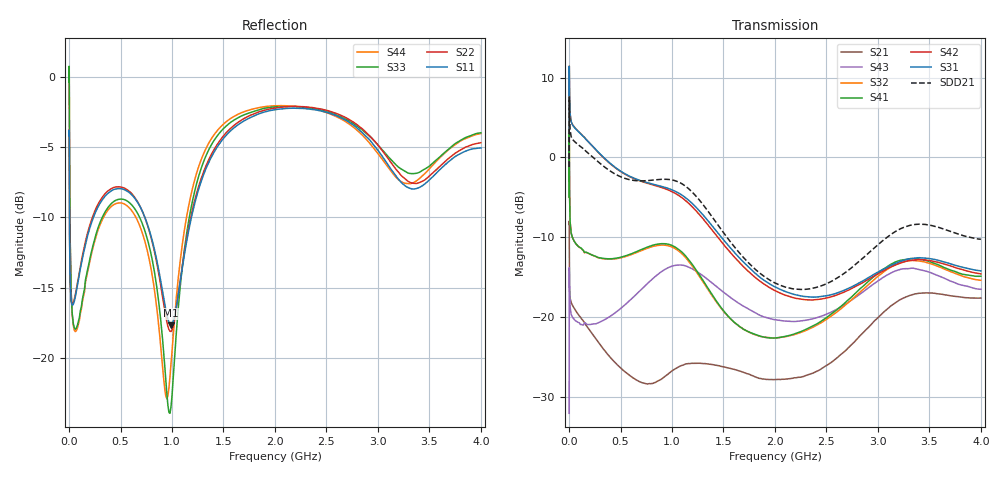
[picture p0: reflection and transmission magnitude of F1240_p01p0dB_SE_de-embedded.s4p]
! Integrated Device Technology
! Corporate Headquarters
! 6024 Silver Creek Valley Road
! San Jose, CA 95138  USA
! Phone:  1-408-284-8200
! Toll Free:  1-800-223-1366
! Webpage:  http://www.idt.com/
! Timing and RF Division
! 515 Groton Road, Suite 102
! Westford, MA 01886-6024
! Device:  F1240
! Description: Dual Intermediate Frequency Digital Variable Gain Amplifier
! Frequency:  10.0 -  500.00 MHz
! Package:  5x5 mm QFN Plastic Package: 32 pin
! Ports:  8 RF, 20 DC
!  Pin  1  = GA3 / Data  Pin 17  = RF OUT_B+
!  Pin  2  = GA4 / CLK  Pin 18  = RF OUT_B-
!  Pin  3  = GA5  Pin 19  = STBY_B
!  Pin  4  = VMODE  Pin 20  = Ground
!  Pin  5  = No Connect  Pin 21  = Ground
!  Pin  6  = GB5  Pin 22  = STB_A
!  Pin  7  = GB4  Pin 23  = RF OUT_A-  = Port 4
!  Pin  8  = GB3  Pin 24  = RF OUT_A+  = Port 3
!  Pin  9  = GB2  Pin 25  = GA0
!  Pin 10  = GB1  Pin 26  = ISET_A
!  Pin 11  = RF IN_B+  Pin 27  = VCC
!  Pin 12  = RF IN_B-  Pin 28  = Ground
!  Pin 13  = Ground  Pin 29  = RF IN_A-  = Port 2
!  Pin 14  = VCC  Pin 30  = RF IN_A+  = Port 1
!  Pin 15  = ISET_B  Pin 31  = GA1
!  Pin 16  = GB0  Pin 32  = GA2 / CSb
! Gain  = +19.5 dB
! State  = 1
! Voltage  = +5.00 V
! Current  = 85.292 mA (one channel only)
! Temperture  =  +25 C
! Test Date  =  2017-10-18
! Board  =  EB4031
! Data:  The device was measured on a custom evaluation board which has
!  individual transmission lines to the RF pins.  Data was collected
!  using a calibrated network analyzer.  The evaluation board was
!  de-embedded using Automatic Fixture Removal.
!  The reference plane is the edge of the package pin.
!  Only Channel A was measured.
!  This data is in single-ended operation.  If your needs are balanced
!  or differential S-parameters then this file needs to be used a
!  linear simulator.
! File Date:  2017-11-10  MJV
! Note:
!  Integrated Device Technology supplies this data as a sample of measured
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# Hz S dB R 100
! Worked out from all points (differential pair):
!   410 points, 500 kHz to 4 GHz, reference 100 ohm
!   strongest paths, dB at 500 kHz, 930 MHz, 1.96 GHz, 2.98 GHz, 4 GHz:
!     S31: 3.1, -3.7, -15.9, -14.5, -14.2
!     S42: 3.1, -3.9, -16.4, -14.7, -14.6
!     S41: -5.0, -10.8, -22.6, -14.7, -14.9
!     S32: -5.0, -11.0, -22.6, -15.1, -15.4
!     S43: -32.0, -14.0, -20.2, -15.7, -16.5
!     S21: -8.4, -27.4, -27.8, -20.3, -17.6
!   taken as a pair (ports 1,2 in; 3,4 out), SDD21 dB: -1.2, -2.7, -15.4, -11.2, -10.3
!   lowest |S11| = -17.7 dB at 990 MHz (marker M1), VSWR 1.30, Z = 78.3 - j8.61 ohm
!   |S11| at or under -10 dB: 4.074 MHz to 236.6 MHz (232.5 MHz wide, 193 % of centre); 736.5 MHz to 1.188 GHz (451.9 MHz wide, 47 % of centre)
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500000  -4.16 -5.5  -8.37 -5.8  -29.56 81.5  -38.35 79.2
        -8.38 -5.7  -4.16 -5.5  -38.33 78.1  -29.56 82.6
        3.15 -106.7  -4.95 -108.1  -0.37 1.0  -32.07 -48.0
        -4.97 -107.0  3.14 -105.5  -32.05 -48.4  -0.37 3.3
2500000  -6.61 -45.4  -12.05 -44.5  -19.08 26.7  -29.60 0.5
         -12.06 -44.5  -6.58 -45.5  -29.55 0.2  -19.08 26.9
         10.77 178.9  1.49 157.6  -1.00 -55.5  -13.81 -151.6
         1.45 157.7  10.76 179.1  -13.79 -151.6  -1.06 -55.2
4500000  -10.67 -50.4  -15.92 -35.4  -19.14 11.0  -32.37 -14.2
         -15.93 -35.4  -10.63 -50.7  -32.34 -14.4  -19.14 11.1
         8.09 162.5  -3.82 140.5  -5.17 -80.6  -16.08 177.6
         -3.87 140.6  8.09 162.7  -16.05 177.5  -5.22 -80.6
1.7e8  -11.59 -109.8  -21.09 -52.5  -21.22 -44.6  -36.04 -21.8
       -21.10 -52.5  -11.38 -111.2  -36.13 -21.3  -21.23 -44.9
       2.19 116.4  -11.91 82.5  -14.08 -135.1  -20.94 108.6
       -11.89 82.4  2.19 115.6  -20.89 108.3  -14.22 -134.7
5.2e8  -7.97 -164.1  -26.61 -106.0  -22.84 -109.0  -33.20 -71.6
       -26.59 -105.2  -7.86 -165.7  -33.36 -69.5  -23.02 -109.5
       -1.88 25.2  -12.52 -42.9  -8.70 -170.3  -18.89 11.7
       -12.44 -44.0  -1.93 24.0  -18.72 11.6  -8.99 -170.8
9.9e8  -17.68 -155.6  -27.13 -142.5  -21.86 150.2  -30.38 -162.9
       -26.83 -145.1  -18.12 -153.3  -30.42 -156.9  -22.43 148.8
       -4.01 -89.8  -11.17 170.9  -23.51 -133.8  -13.91 -111.6
       -10.97 167.3  -4.23 -92.4  -13.66 -111.8  -20.43 -114.3
4e9  -5.05 -140.9  -17.65 104.5  -24.07 -44.2  -25.04 -27.8
     -17.62 104.3  -4.67 -139.2  -25.91 -12.3  -25.80 -37.4
     -14.21 39.8  -15.39 -65.0  -3.96 -134.5  -18.00 66.9
     -14.88 -78.6  -14.58 45.8  -16.52 57.8  -4.02 -144.2
